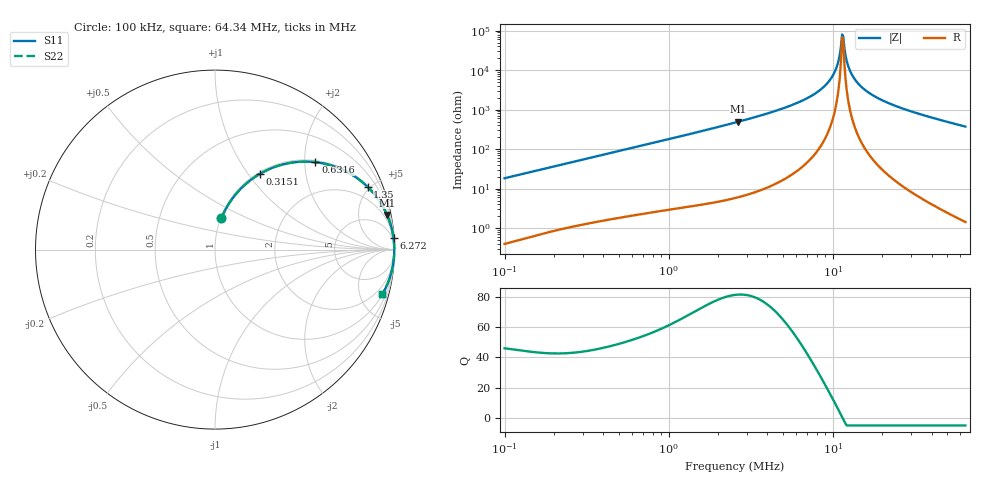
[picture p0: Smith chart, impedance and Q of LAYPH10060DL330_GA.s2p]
! LAYPH10060DL330_GA  S-PARAMETER MODEL  ( General Type )
! Model Generated by TAIYO YUDEN Corporation (http://www.ty-top.com)
! Version 3.0
! TAIYO YUDEN Control No. 180828NI43SB-FBB
! Copyright(c) 2017 TAIYO YUDEN CO.,LTD. All Rights Reserved.
! Product Description (link to TY-COMPAS)
! https://ds.yuden.co.jp/TYCOMPAS/or/detail?pn=LAYPH10060DL330MGA&u=M
! Products Name : Inductors
! Characteristics :
!  Inductance : 33 uH , SRF(min) : -Hz , DC Resistance(max) : 0.073 Ohm
!  Rated Current : Saturation :2.4 A , Temp Rise : 1.8 A (25 degC)
!  Case Size : 10.1 x 10.0 / 0.398 x 0.394 [mm/inch] , Thickness : 6 / 0.236 [mm/inch]
!  (Conditions: Temperature = 25 degC , DC Bias Current/Voltage = 0A / 0V)
! External Node Assignments :
!  1  o---GGG---o  2
! GND o---------o GND
! Frequency Range : 0.1MHz  -  64.339822MHz  [ 402 STEP ]
# MHz S RI R 50
! Freq[MHz].  S11 Real  S11 Imag  S21 Real  S21 Imag  S12 Real  S12 Imag  S22 Real  S22 Imag
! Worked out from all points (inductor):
!   401 points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, 100 kHz to 64.34 MHz, reference 50 ohm
!   read as one part in series: L = 29.1 uH near 103.3 kHz
!   highest Q = 81.6 at 2.663 MHz (marker M1), where L = 29.6 uH
!   self-resonance near 11.41 MHz
!   S11 on the Smith chart (normalised r, x): 100 kHz: 1.01, +0.37; 315.1 kHz: 1.03, +1.14; 631.6 kHz: 1.04, +2.26; 1.35 MHz: 1.07, +4.84; 6.272 MHz: 2, +31; 64.34 MHz: 1.03, -7.45
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0.1  0.0361 0.1761  0.9639 -0.1761  0.9639 -0.1761  0.0361 0.1761
0.295407  0.2263 0.4072  0.7737 -0.4072  0.7737 -0.4072  0.2263 0.4072
0.315141  0.2487 0.4211  0.7513 -0.4211  0.7513 -0.4211  0.2487 0.4211
0.631563  0.5592 0.487  0.4408 -0.487  0.4408 -0.487  0.5592 0.487
0.872651  0.7051 0.4475  0.2949 -0.4475  0.2949 -0.4475  0.7051 0.4475
1.350247  0.8507 0.3492  0.1493 -0.3492  0.1493 -0.3492  0.8507 0.3492
2.53653  0.9544 0.2025  0.0456 -0.2025  0.0456 -0.2025  0.9544 0.2025
2.662585  0.9588 0.1928  0.0412 -0.1928  0.0412 -0.1928  0.9588 0.1928
6.272304  0.9947 0.0631  0.00527 -0.0631  0.00527 -0.0631  0.9947 0.0631
7.493079  0.9969 0.0433  0.00306 -0.0433  0.00306 -0.0433  0.9969 0.0433
8.807898  0.9982 0.0265  0.00183 -0.0265  0.00183 -0.0265  0.9982 0.0265
9.863265  0.9987 0.0151  0.00132 -0.0151  0.00132 -0.0151  0.9987 0.0151
10.52217  0.9988 0.00864  0.00116 -0.00864  0.00116 -0.00864  0.9988 0.00864
11.2251  0.9989 0.00224  0.00107 -0.00224  0.00107 -0.00224  0.9989 0.00224
11.40805  0.9989 0.000645  0.00107 -0.000645  0.00107 -0.000645  0.9989 0.000645
11.78295  0.9989 -0.00255  0.00107 0.00255  0.00107 0.00255  0.9989 -0.00255
12.17016  0.9989 -0.00574  0.00109 0.00574  0.00109 0.00574  0.9989 -0.00574
12.77497  0.9988 -0.0105  0.00116 0.0105  0.00116 0.0105  0.9988 -0.0105
14.07625  0.9986 -0.0202  0.00145 0.0202  0.00145 0.0202  0.9986 -0.0202
16.81591  0.9975 -0.0385  0.00251 0.0385  0.00251 0.0385  0.9975 -0.0385
22.13506  0.9942 -0.0692  0.00583 0.0692  0.00583 0.0692  0.9942 -0.0692
64.33982  0.932 -0.2499  0.068 0.2499  0.068 0.2499  0.932 -0.2499
